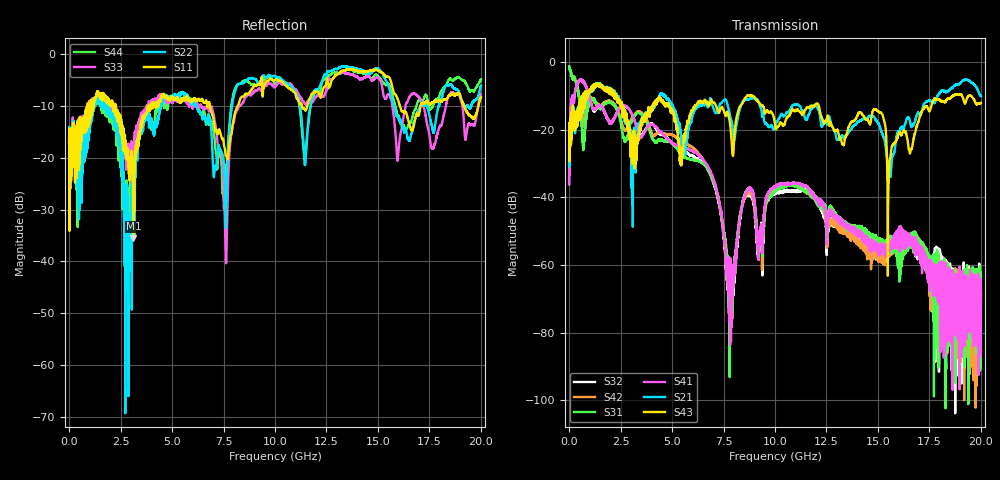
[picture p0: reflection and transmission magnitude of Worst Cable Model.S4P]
! The contents of this file provide the 4 port S-parameters for
! the Worst Cable Emulator referenced in the HDMI 2.0 Specification,
! Section 6.1.1.4
! Copyright (C) 2013 HDMI Forum, All Rights Reserved.
! THE CONTENTS OF THIS FILE ARE PROVIDED "AS IS", WITHOUT WARRANTY OF ANY KIND,
! EXPRESS OR IMPLIED, INCLUDING BUT NOT LIMITED TO THE WARRANTIES OF
! MERCHANTABILITY, FITNESS FOR A PARTICULAR PURPOSE, TITLE AND NON-INFRINGEMENT.
! IN NO EVENT SHALL THE COPYRIGHT HOLDERS BE LIABLE FOR ANY DAMAGES OR OTHER
! LIABILITY, WHETHER IN CONTRACT, TORT OR OTHERWISE, ARISING FROM, OUT OF OR IN
! CONNECTION WITH THE CONTENTS OF THIS FILE.
!Data & Calibration Information:
!Freq	S11:SOLT4(ON)	S12:SOLT4(ON)	S13:SOLT4(ON)	S14:SOLT4(ON)
!	S21:SOLT4(ON)	S22:SOLT4(ON)	S23:SOLT4(ON)	S24:SOLT4(ON)
!	S31:SOLT4(ON)	S32:SOLT4(ON)	S33:SOLT4(ON)	S34:SOLT4(ON)
!	S41:SOLT4(ON)	S42:SOLT4(ON)	S43:SOLT4(ON)	S44:SOLT4(ON)
!PortZ  Port1:50+j0  Port2:50+j0  Port3:50+j0  Port4:50+j0
!Above PortZ is port z conversion or system Z0 setting when saving the data.
!When reading, reference impedance value at option line is always used.
# Hz S MA R 50
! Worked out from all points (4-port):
!   20000 points, 1 MHz to 20 GHz, reference 50 ohm
!   strongest paths, dB at 1 MHz, 5.001 GHz, 10 GHz, 15 GHz, 20 GHz:
!     S43: -29.2, -14.1, -18.4, -14.6, -12.0
!     S21: -29.1, -12.6, -19.0, -18.0, -10.0
!     S41: -36.1, -24.0, -36.7, -55.9, -73.6
!     S31: -1.2, -24.1, -38.2, -53.3, -62.4
!     S42: -1.2, -21.6, -38.0, -55.9, -70.8
!     S32: -36.0, -23.9, -38.7, -54.3, -69.0
!   lowest |S11| = -35.6 dB at 3.125 GHz (marker M1), VSWR 1.03, Z = 50.9 - j1.42 ohm
!   |S11| at or under -10 dB: 2.252 GHz to 3.88 GHz (1.628 GHz wide, 53.1 % of centre); 6.833 GHz to 8.184 GHz (1.352 GHz wide, 18 % of centre); 16.07 GHz to 17.07 GHz (1.001 GHz wide, 6.04 % of centre)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
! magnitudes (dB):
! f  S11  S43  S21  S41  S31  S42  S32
! 1 MHz  -17.0  -29.2  -29.1  -36.1  -1.2  -1.2  -36.0
! 3.125 GHz  -35.6  -21.1  -25.2  -16.5  -16.3  -15.9  -16.4
! 6.768 GHz  -9.3  -12.5  -12.9  -31.1  -32.1  -31.3  -32.1
! 7.89 GHz  -15.4  -23.0  -17.3  -63.2  -76.3  -65.4  -61.1
! 8.575 GHz  -7.7  -10.4  -11.0  -39.1  -38.7  -39.5  -39.7
! 10.73 GHz  -6.7  -15.3  -14.0  -36.0  -36.5  -36.0  -38.0
! 20 GHz  -8.3  -12.0  -10.0  -73.6  -62.4  -70.8  -69.0
